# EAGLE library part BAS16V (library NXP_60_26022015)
High-speed switching diodes High-speed switching diodes, encapsulated in small Surface-Mounted Device (SMD) plastic packages. AAL Eindhoven MK
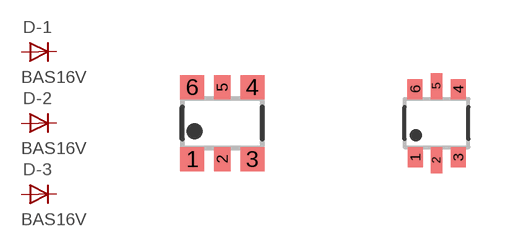
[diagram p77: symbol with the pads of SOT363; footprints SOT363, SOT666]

Designator prefix D; gates -1=DIODE -2=DIODE -3=DIODE

## BAS16VY  [SOT363]
1  -1:A  pas
2  -2:A  pas
3  -3:A  pas
4  -3:K  pas
5  -2:K  pas
6  -1:K  pas

## BAS16VV  [SOT666]
Pads as for SOT363

## Footprint SOT363 (pad centres in mm)
SOT363 Plastic surface-mounted package; 6 leads JEDEC: -- IEC: -- JEITA: SC-88
smd 0.6 x 0.6: 1 -0.75,-0.9; 3 0.75,-0.9; 4 0.75,0.9; 6 -0.75,0.9
smd 0.4 x 0.6: 2 0,-0.9; 5 0,0.9

## Footprint SOT666 (pad centres in mm)
SOT 666 Reflow soldering foorprint Source: Philips - BAS70_1PS7XSB70_SER_8.pdf
smd 0.375 x 0.5: 1 -0.537,-0.85; 3 0.538,-0.85; 4 0.538,0.85; 6 -0.538,0.85
smd 0.3 x 0.65: 2 0,-0.925; 5 0,0.925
